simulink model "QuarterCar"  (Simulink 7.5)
settings: Solver=ode45  StartTime=0.0  StopTime=5  FixedStep=0.001  MaxStep=Ts  RelTol=1e-3
PreLoadFcn:
  | QuarterCarParams
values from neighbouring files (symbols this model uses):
  actuatorDelay = 0.005    [QuarterCarParams.m]
  actuatorPole = 70    [QuarterCarParams.m]
  actuatorSat = 4000    [QuarterCarParams.m]
  g = 9.81    [QuarterCarParams.m]
  J = 1    [QuarterCarParams.m]
  Ki = 100000    [QuarterCarParams.m]
  Kp = 1200    [QuarterCarParams.m]
  lambda_ref = 0.1    [QuarterCarParams.m]
  m = 450    [QuarterCarParams.m]
  roadCoeffs = [1.28 23.99 0.52]    [QuarterCarParams.m]
  Ts = 0.005    [QuarterCarParams.m]
  v0 = 30    [QuarterCarParams.m]
  Wr = 0.32    [QuarterCarParams.m]
undefined symbols (not defined in the file or in its folder): DiscIntNeverNeededParam
libraries: simulink x1

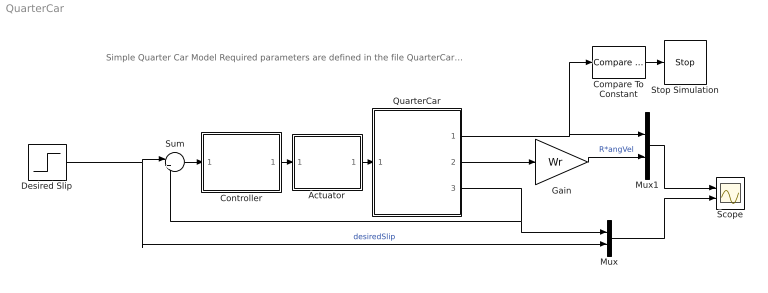
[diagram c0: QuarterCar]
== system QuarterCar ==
  note: Simple Quarter Car Model Required parameters are defined in the file QuarterCarParams.m
  Actuator : Subsystem  TreatAsAtomicUnit=on
  Compare To Constant : simulink/Logic and Bit Operations/Compare To Constant  SystemSampleTime=-1  relop=<  const=0.5  LogicOutDataTypeMode=boolean
  Controller : Subsystem  TreatAsAtomicUnit=on  SystemSampleTime=Ts
  Desired Slip : Step  Time=0.2  After=lambda_ref  SampleTime=0
  Gain : Gain  Gain=Wr  ParameterDataType=fixdt(1, 16)  ParameterScaling=2^0  OutDataType=fixdt(1, 16)  OutScaling=2^0
  Mux : Mux  Inputs=2
  Mux1 : Mux  Inputs=2
  QuarterCar : Subsystem  TreatAsAtomicUnit=on
  Scope : Scope  NumInputPorts=2
  Stop Simulation : Stop
  Sum : Sum  Inputs=|+-  OutDataType=sfix(16)  OutScaling=2^0
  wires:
  Controller/1(u) -> Actuator/1(Tb_ref)
  Sum/1 -> Controller/1(slip_error)
  Actuator/1(Tb) -> QuarterCar/1(Tb)
  Desired Slip/1 -> Sum/1, Mux/2  "desiredSlip"
  QuarterCar/3(lambda) -> Mux/1, Sum/2
  QuarterCar/1(vel) -> Mux1/1, Compare To Constant/1
  QuarterCar/2(angVel) -> Gain/1
  Mux1/1 -> Scope/1
  Mux/1 -> Scope/2
  Gain/1 -> Mux1/2  "R*angVel"
  Compare To Constant/1 -> Stop Simulation/1

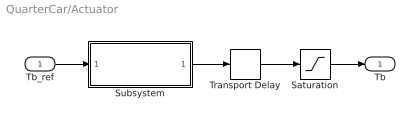
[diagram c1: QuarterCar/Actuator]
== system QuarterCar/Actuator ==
  Tb_ref : Inport
  Saturation : Saturate  UpperLimit=actuatorSat  LowerLimit=0
  Subsystem : Subsystem
  Transport Delay : TransportDelay  DelayTime=actuatorDelay  BufferSize=10240
  Tb : Outport
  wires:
  Subsystem/1(Tb) -> Transport Delay/1
  Tb_ref/1 -> Subsystem/1(Tb_ref)
  Saturation/1 -> Tb/1
  Transport Delay/1 -> Saturation/1

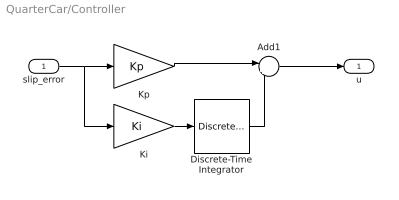
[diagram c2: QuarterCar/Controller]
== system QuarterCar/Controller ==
  slip_error : Inport  OutDataType=sfix(16)  OutScaling=2^0
  Add1 : Sum  Inputs=|++  OutDataType=sfix(16)  OutScaling=2^-10
  Discrete-Time Integrator : DiscreteIntegrator  SampleTime=-1  OutDataType=fixdt(1, 16)  OutScaling=2^0  ICPrevOutput=DiscIntNeverNeededParam  ICPrevScaledInput=DiscIntNeverNeededParam
  Ki : Gain  Gain=Ki  ParameterDataType=sfix(16)  ParameterScaling=2^0  OutDataType=sfix(16)  OutScaling=2^0
  Kp : Gain  Gain=Kp  ParameterDataType=sfix(16)  ParameterScaling=2^0  OutDataType=sfix(16)  OutScaling=2^0
  u : Outport  OutDataType=sfix(16)  OutScaling=2^0
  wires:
  slip_error/1 -> Kp/1, Ki/1
  Add1/1 -> u/1
  Kp/1 -> Add1/1
  Ki/1 -> Discrete-Time Integrator/1
  Discrete-Time Integrator/1 -> Add1/2

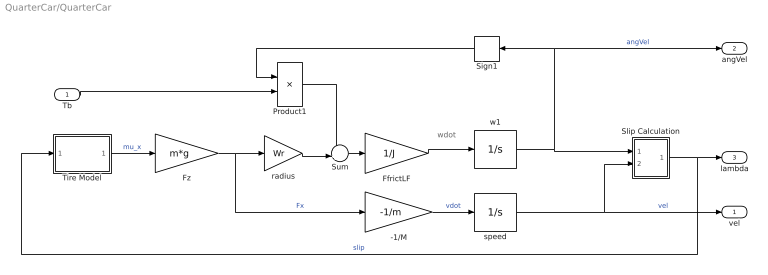
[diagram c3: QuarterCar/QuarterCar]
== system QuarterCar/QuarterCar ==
  note: wdot
  Tb : Inport  OutDataType=sfix(16)  OutScaling=2^0
  -1/M : Gain  Gain=-1/m  ParameterDataType=sfix(16)  ParameterScaling=2^0  OutDataType=sfix(16)  OutScaling=2^0
  FfrictLF : Gain  Gain=1/J  ParameterDataType=sfix(16)  ParameterScaling=2^0  OutDataType=sfix(16)  OutScaling=2^0
  Fz : Gain  Gain=m*g  ParameterDataType=sfix(16)  ParameterScaling=2^0  OutDataType=sfix(16)  OutScaling=2^0
  Product1 : Product  OutDataType=sfix(16)  OutScaling=2^0
  Sign1 : Signum
  Slip Calculation : Subsystem
  Sum : Sum  Inputs=-+|  OutDataType=sfix(16)  OutScaling=2^0
  Tire Model : Subsystem  TreatAsAtomicUnit=on
  radius : Gain  Gain=Wr  ParameterDataType=sfix(16)  ParameterScaling=2^0  OutDataType=sfix(16)  OutScaling=2^0
  speed : Integrator  InitialCondition=v0  LimitOutput=on  LowerSaturationLimit=0
  w1 : Integrator  InitialCondition=v0/Wr  LimitOutput=on  LowerSaturationLimit=0
  vel : Outport  OutDataType=sfix(16)  OutScaling=2^0
  angVel : Outport  Port=2  OutDataType=sfix(16)  OutScaling=2^0
  lambda : Outport  Port=3  OutDataType=sfix(16)  OutScaling=2^0
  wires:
  -1/M/1 -> speed/1  "vdot"
  Fz/1 -> -1/M/1, radius/1  "Fx"
  Slip Calculation/1(slip) -> lambda/1, Tire Model/1(slip)  "slip"
  FfrictLF/1 -> w1/1
  Sign1/1 -> Product1/1
  Tb/1 -> Product1/2
  w1/1 -> Sign1/1, angVel/1, Slip Calculation/1(w)  "angVel"
  speed/1 -> Slip Calculation/2(v), vel/1  "vel"
  Sum/1 -> FfrictLF/1
  Tire Model/1(mu_x) -> Fz/1  "mu_x"
  radius/1 -> Sum/2
  Product1/1 -> Sum/1

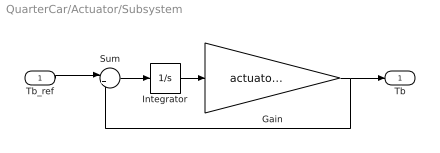
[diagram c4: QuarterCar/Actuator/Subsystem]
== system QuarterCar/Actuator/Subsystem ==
  Tb_ref : Inport  OutDataType=fixdt(1, 16)  OutScaling=2^0
  Gain : Gain  Gain=actuatorPole  ParameterDataType=fixdt(1, 16)  ParameterScaling=2^0  OutDataType=fixdt(1, 16)  OutScaling=2^0
  Integrator : Integrator
  Sum : Sum  Inputs=|+-  OutDataType=fixdt(1, 16)  OutScaling=2^0
  Tb : Outport  OutDataType=fixdt(1, 16)  OutScaling=2^0
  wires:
  Gain/1 -> Tb/1, Sum/2
  Tb_ref/1 -> Sum/1
  Sum/1 -> Integrator/1
  Integrator/1 -> Gain/1

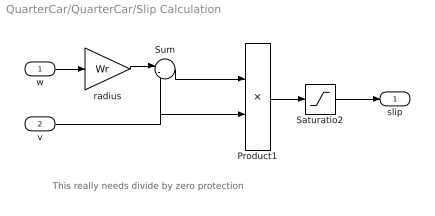
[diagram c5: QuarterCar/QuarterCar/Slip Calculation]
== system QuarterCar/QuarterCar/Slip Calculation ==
  note: This really needs divide by zero protection
  w : Inport  OutDataType=fixdt(1, 16)  OutScaling=2^0
  v : Inport  Port=2  OutDataType=fixdt(1, 16)  OutScaling=2^0
  Product1 : Product  Inputs=*/  OutDataType=sfix(16)  OutScaling=2^0
  Saturatio2 : Saturate  UpperLimit=1  LowerLimit=0
  Sum : Sum  Inputs=|-+  OutDataType=sfix(16)  OutScaling=2^0
  radius : Gain  Gain=Wr  ParameterDataType=sfix(16)  ParameterScaling=2^0  OutDataType=sfix(16)  OutScaling=2^0
  slip : Outport  OutDataType=fixdt(1, 16)  OutScaling=2^0
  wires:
  w/1 -> radius/1
  v/1 -> Sum/2, Product1/2
  radius/1 -> Sum/1
  Sum/1 -> Product1/1
  Product1/1 -> Saturatio2/1
  Saturatio2/1 -> slip/1

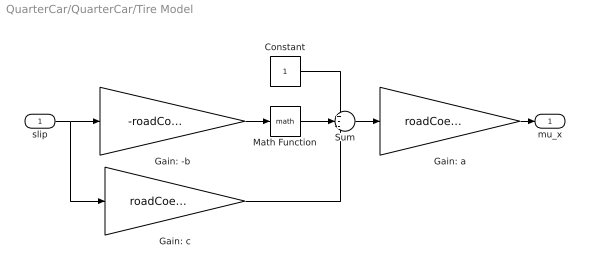
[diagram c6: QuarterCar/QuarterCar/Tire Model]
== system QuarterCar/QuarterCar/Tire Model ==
  slip : Inport  OutDataType=fixdt(1, 16)  OutScaling=2^0
  Constant : Constant  OutDataType=fixdt(1, 16)  OutScaling=2^0
  Gain: -b : Gain  Gain=-roadCoeffs(2)  ParameterDataType=sfix(16)  ParameterScaling=2^0  OutDataType=sfix(16)  OutScaling=2^0
  Gain: a : Gain  Gain=roadCoeffs(1)  ParameterDataType=sfix(16)  ParameterScaling=2^0  OutDataType=sfix(16)  OutScaling=2^0
  Gain: c : Gain  Gain=roadCoeffs(3)  ParameterDataType=sfix(16)  ParameterScaling=2^0  OutDataType=sfix(16)  OutScaling=2^0
  Math Function : Math  OutDataType=fixdt(1, 16)  OutScaling=2^0
  Sum : Sum  Inputs=+--  OutDataType=fixdt(1, 16)  OutScaling=2^0
  mu_x : Outport  OutDataType=fixdt(1, 16)  OutScaling=2^0
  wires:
  slip/1 -> Gain: -b/1, Gain: c/1
  Gain: -b/1 -> Math Function/1
  Math Function/1 -> Sum/2
  Constant/1 -> Sum/1
  Gain: c/1 -> Sum/3
  Sum/1 -> Gain: a/1
  Gain: a/1 -> mu_x/1
